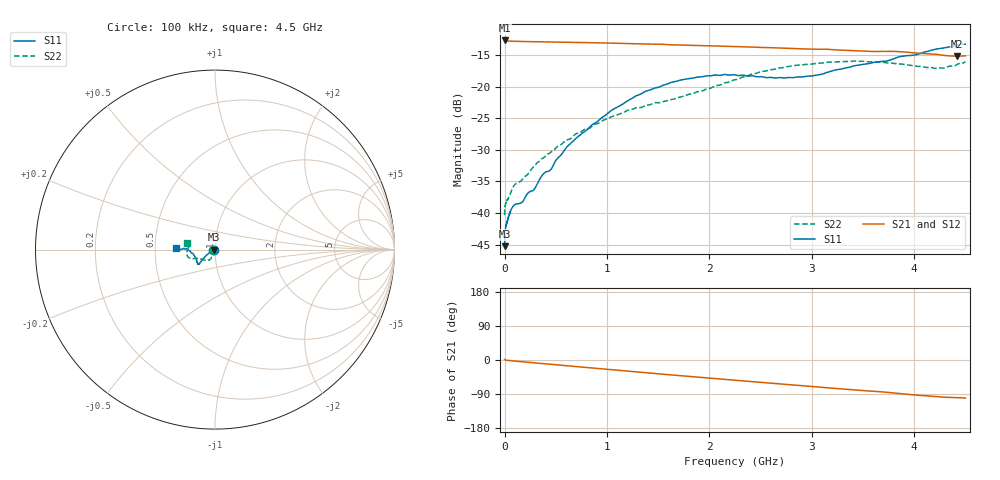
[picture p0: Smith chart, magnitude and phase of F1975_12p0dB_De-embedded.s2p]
! Integrated Device Technology
! Corporate Headquarters
! 6024 Silver Creek Valley Road
! San Jose, CA 95138  USA
! Phone:  1-408-284-8200
! Toll Free:  1-800-223-1366
! Webpage:  http://www.idt.com/
! Timing and RF Division
! 515 Groton Road, Suite 102
! Westford, MA 01886-6024
! Device:  F1975
! Description: 6-bit, 75 ohm, 0.5 dB Digital Step Attenuator
! Frequency:  5.0 MHz -  3.00 GHz
! Package:  4x4 mm QFN Plastic Package: 20 pin
! Ports:  2 RF, 11 DC
!  Pin  1  = D5 (16 dB)
!  Pin  2  = RF1  =  Port 1
!  Pin  3  = Serial Data In (DATA)
!  Pin  4  = Serial Clock (CLK)
!  Pin  5  = Serial Latch Enable (LE)
!  Pin  6  = VDD
!  Pin  7  = NC
!  Pin  8  = NC
!  Pin  9  = NC
!  Pin 10  = GND
!  Pin 11  = GND
!  Pin 12  = NC
!  Pin 13  = VMODE
!  Pin 14  = RF2  =  Port 2
!  Pin 15  = D4 (8 dB)
!  Pin 16  = D3 (4 dB)
!  Pin 17  = D2 (2 dB)
!  Pin 18  = NC
!  Pin 19  = D1 (1 dB)
!  Pin 20  = D0 (0.5 dB)
! State:  24
! Atten State:  12.0 dB
! Voltage:  +3.30 Volts
! Current:  0.595 mA
! Data:  The device was measured on a F1975 evaluation board which has
!  individual transmission lines to the RF pins.  Data was collected
!  using a calibrated network analyzer.  The evaluation board was
!  de-embedded using Automatic Fixture Removal (AFR).
!  The reference plane is the edge of the package pin.
! Misc:
!  Action Tracker AT0415
! Date Measured:  2018-02-08
! Date:  2018-03-26  MJV
! Note:
!  Integrated Device Technology supplies this data as a sample of measured
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# GHz S dB R 75
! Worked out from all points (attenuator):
!   291 points, 100 kHz to 4.5 GHz, reference 75 ohm
!   highest |S21| = -12.64 dB at 100 kHz (marker M1); lowest = -15.1 dB at 4.42 GHz (marker M2)
!   lowest |S11| = -45.3 dB at 100 kHz (marker M3), VSWR 1.01, Z = 74.2 + j0.00614 ohm
!   |S11| at or under -10 dB: start of sweep to end of sweep
!   |S22| runs from -40.3 to -15.9 dB; largest |S21 - S12| = 0.00014
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0.0001  -45.25 179.6  -12.64 1.2  -12.64 1.2  -40.33 -177.4
0.0005  -43.96 -175.6  -12.66 1.1  -12.66 1.1  -39.77 -176.3
0.002  -43.34 -174.8  -12.68 0.8  -12.68 0.9  -39.23 -175.5
0.012  -42.08 -171.5  -12.71 -0.5  -12.71 -0.5  -38.40 -170.9
0.08  -38.99 -161.2  -12.76 -2.3  -12.76 -2.3  -35.94 -156.0
0.18  -38.16 -156.4  -12.81 -4.8  -12.80 -4.8  -34.52 -135.8
0.22  -36.97 -156.4  -12.82 -5.8  -12.82 -5.8  -33.96 -130.5
0.28  -36.44 -153.8  -12.84 -7.3  -12.83 -7.2  -32.70 -127.5
0.36  -34.18 -154.9  -12.86 -9.2  -12.86 -9.2  -31.43 -120.4
0.44  -33.28 -152.0  -12.88 -11.1  -12.88 -11.1  -30.51 -115.6
0.6  -29.67 -152.6  -12.93 -15.0  -12.92 -15.0  -28.45 -114.0
0.76  -27.33 -148.2  -12.97 -18.8  -12.97 -18.8  -26.97 -113.7
1.06  -23.56 -144.6  -13.07 -26.0  -13.07 -26.0  -24.63 -115.6
1.52  -19.96 -139.8  -13.25 -36.7  -13.24 -36.7  -22.50 -127.3
1.88  -18.46 -137.9  -13.44 -45.0  -13.44 -45.0  -20.78 -142.5
2.26  -18.13 -141.1  -13.61 -53.6  -13.60 -53.6  -18.83 -154.0
2.68  -18.52 -154.7  -13.83 -62.9  -13.83 -62.9  -17.01 -158.9
3.02  -18.21 -168.1  -14.02 -70.2  -14.02 -70.2  -16.33 -163.1
3.76  -15.77 178.9  -14.36 -85.9  -14.36 -85.9  -16.22 -178.3
4.2  -14.06 179.7  -14.82 -96.2  -14.82 -96.2  -17.07 169.8
4.42  -13.35 -179.9  -15.14 -99.4  -15.14 -99.4  -16.42 166.7
4.5  -13.23 178.3  -15.08 -100.6  -15.07 -100.6  -16.00 165.6
